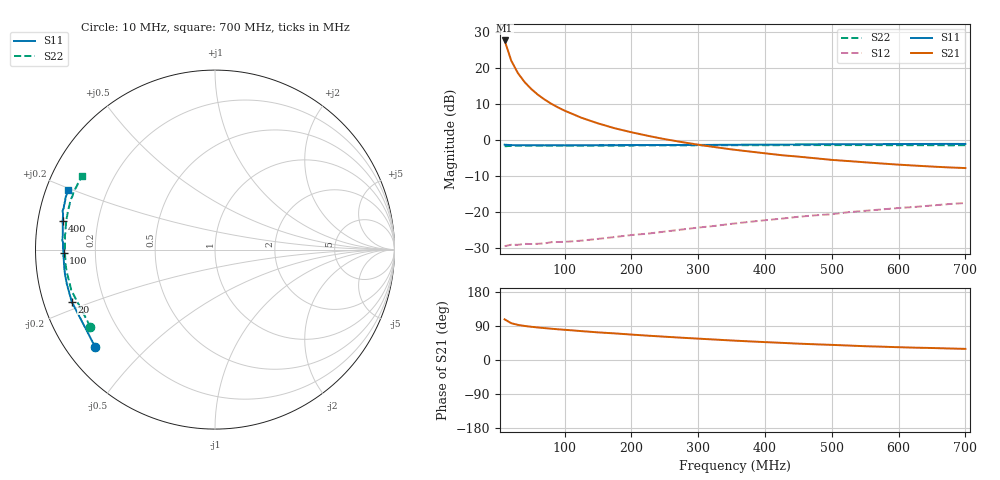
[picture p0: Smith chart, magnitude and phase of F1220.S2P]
! Date: Mon Aug 07 16:12:55 1995
# MHZ  S  MA  R  50.0000
!  POLYFET RF DEVICES
!  F1220
!  S PARAMETERS
!  VDS=12.5V, IDQ=400mA
!FREQ  S11MAG S11ANG S21MAG S21ANG S12MAG S12ANG S22MAG S22ANG
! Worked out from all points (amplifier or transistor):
!   34 points, 10 MHz to 700 MHz, reference 50 ohm
!   highest |S21| = 27.6 dB at 10 MHz (marker M1)
!   |S21| within 3 dB of that: start of sweep to 15.32 MHz
!   unconditionally stable (mu >= 1): 202.7 MHz to end of sweep
!   at 60 MHz: K = 0.41, MSG = 20.7 dB, |S12| = -28.8 dB
!   at 300 MHz: K = 1.13, MAG = 9.3 dB, |S12| = -24.3 dB
!   at 700 MHz: K = 1.07, MAG = 3.2 dB, |S12| = -17.5 dB
!   S11 on the Smith chart (normalised r, x): 10 MHz: 0.08, -0.35; 20 MHz: 0.08, -0.17; 100 MHz: 0.08, -0.01; 400 MHz: 0.07, +0.09; 700 MHz: 0.07, +0.19
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10  0.8609 -140.7  24.03 107.3  0.03369 22.5  0.8166 -148.2
20  0.8494 -160.0  12.56 97.0  0.03528 13.1  0.8321 -164.2
30  0.8475 -167.0  8.449 92.7  0.03517 12.5  0.8334 -170.1
40  0.8469 -170.7  6.35 89.8  0.03626 13.8  0.836 -173.3
50  0.8458 -173.0  5.088 87.7  0.03607 15.2  0.8367 -175.3
60  0.8451 -174.6  4.237 85.8  0.03638 17.0  0.8354 -176.9
70  0.8442 -176.2  3.636 84.1  0.03681 18.4  0.8361 -178.3
80  0.8452 -177.1  3.177 82.5  0.03829 19.3  0.8371 -179.4
90  0.8454 -177.8  2.832 81.0  0.03849 21.1  0.8367 179.9
100  0.8439 -178.6  2.549 79.7  0.03866 23.2  0.8361 179.1
125  0.8463 179.9  2.037 76.2  0.04018 27.8  0.8372 177.4
150  0.847 178.6  1.699 72.9  0.04251 30.4  0.8379 175.8
175  0.8476 177.4  1.455 70.2  0.04511 34.0  0.8402 174.7
200  0.852 176.4  1.28 67.1  0.0481 37.5  0.8381 173.2
225  0.8519 175.4  1.141 64.1  0.05038 39.6  0.8409 172.1
250  0.8518 174.7  1.027 61.5  0.05367 42.3  0.8416 170.8
300  0.8549 172.7  0.8607 56.4  0.06103 45.4  0.8454 168.4
375  0.8621 170.0  0.6955 49.3  0.07298 49.1  0.8475 165.1
400  0.8644 169.2  0.6539 47.2  0.07717 49.2  0.8475 164.0
475  0.8704 166.6  0.5585 41.4  0.0902 50.3  0.8499 160.6
600  0.8787 161.7  0.4552 33.7  0.1139 49.6  0.8471 155.2
700  0.8818 157.9  0.4082 29.4  0.1338 47.8  0.8457 151.0
